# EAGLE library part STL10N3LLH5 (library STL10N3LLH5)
STMICROELECTRONICS - STL10N3LLH5 - MOSFET, N-CH, 30V, 9A, POWERFLAT Source: Datasheet
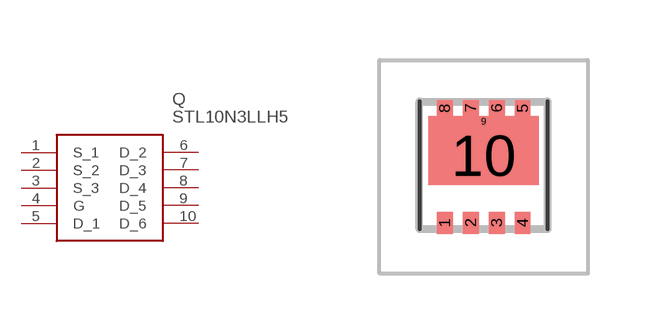
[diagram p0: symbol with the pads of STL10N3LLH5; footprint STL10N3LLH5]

Designator prefix Q

## STL10N3LLH5 (Description: STMICROELECTRONICS - STL10N3LLH5 - MOSFET, N-CH, 30V, 9A, POWERFLAT; Height: 1mm; Manufacturer_Name: STMicroelectronics; Manufacturer_Part_Number: STL10N3LLH5; Mouser_Part_Number: 511-STL10N3LLH5; Mouser_Price-Stock: https://www.mouser.co.uk/ProductDetail/STMicroelectronics/STL10N3LLH5?qs=0gj%2FgiofzsOGxczN3DPYlA%3D%3D)  [STL10N3LLH5]
1  S_1
2  S_2
3  S_3
4  G
5  D_1
6  D_2
7  D_3
8  D_4
9  D_5
10  D_6

## Footprint STL10N3LLH5 (pad centres in mm)
STL10N3LLH5-1
smd 0.4 x 0.55: 1 -0.975,-1.435; 2 -0.325,-1.435; 3 0.325,-1.435; 4 0.975,-1.435
smd 0.4 x 0.41: 5 0.975,1.435; 6 0.325,1.435; 7 -0.325,1.435; 8 -0.975,1.435
smd 2.75 x 0.25: 9 0,1.105
smd 2.75 x 1.47: 10 0,0.245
